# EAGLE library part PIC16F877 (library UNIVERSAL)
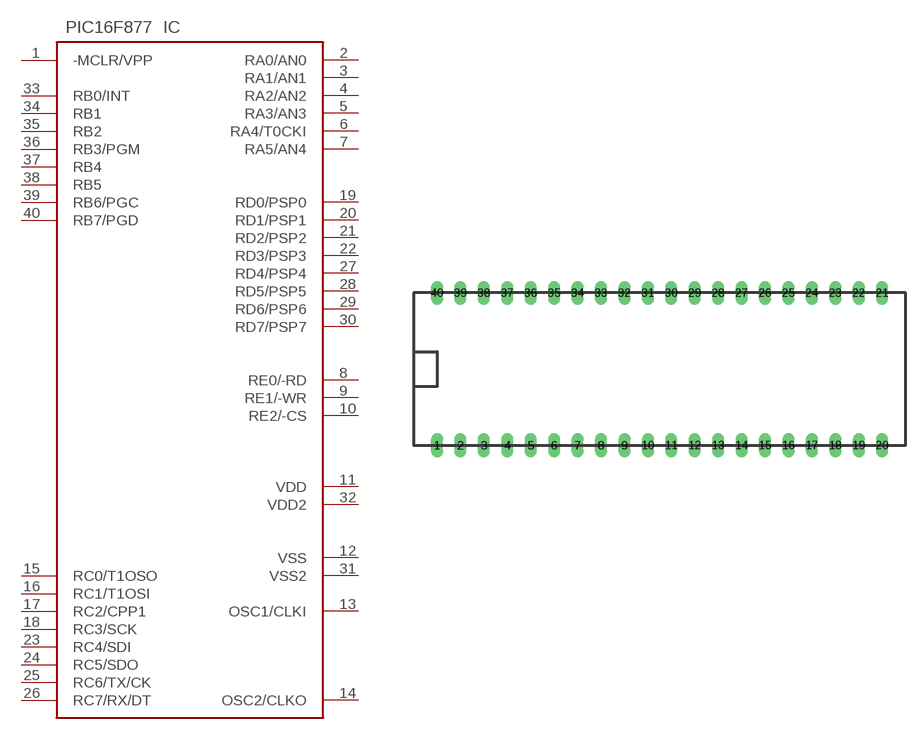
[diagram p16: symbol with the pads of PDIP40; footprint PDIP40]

Designator prefix IC

## PIC16F877  [PDIP40]
1  -MCLR/VPP  in
2  RA0/AN0
3  RA1/AN1
4  RA2/AN2
5  RA3/AN3
6  RA4/T0CKI
7  RA5/AN4
8  RE0/-RD
9  RE1/-WR
10  RE2/-CS
11  VDD  sup
12  VSS  sup
13  OSC1/CLKI  in
14  OSC2/CLKO  out
15  RC0/T1OSO
16  RC1/T1OSI
17  RC2/CPP1
18  RC3/SCK
19  RD0/PSP0
20  RD1/PSP1
21  RD2/PSP2
22  RD3/PSP3
23  RC4/SDI
24  RC5/SDO
25  RC6/TX/CK
26  RC7/RX/DT
27  RD4/PSP4
28  RD5/PSP5
29  RD6/PSP6
30  RD7/PSP7
31  VSS2  sup
32  VDD2  sup
33  RB0/INT
34  RB1
35  RB2
36  RB3/PGM
37  RB4
38  RB5
39  RB6/PGC
40  RB7/PGD

## Footprint PDIP40 (pad centres in mm)
drill 0.813 pad 0.965 long: 1 0,0; 2 2.54,0; 3 5.08,0; 4 7.62,0; 5 10.16,0; 6 12.7,0; 7 15.24,0; 8 17.78,0; 9 20.32,0; 10 22.86,0; 11 25.4,0; 12 27.94,0; 13 30.48,0; 14 33.02,0; 15 35.56,0; 16 38.1,0; 17 40.64,0; 18 43.18,0; 19 45.72,0; 20 48.26,0; 21 48.26,16.51; 22 45.72,16.51; 23 43.18,16.51; 24 40.64,16.51; 25 38.1,16.51; 26 35.56,16.51; 27 33.02,16.51; 28 30.48,16.51; 29 27.94,16.51; 30 25.4,16.51; 31 22.86,16.51; 32 20.32,16.51; 33 17.78,16.51; 34 15.24,16.51; 35 12.7,16.51; 36 10.16,16.51; 37 7.62,16.51; 38 5.08,16.51; 39 2.54,16.51; 40 0,16.51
